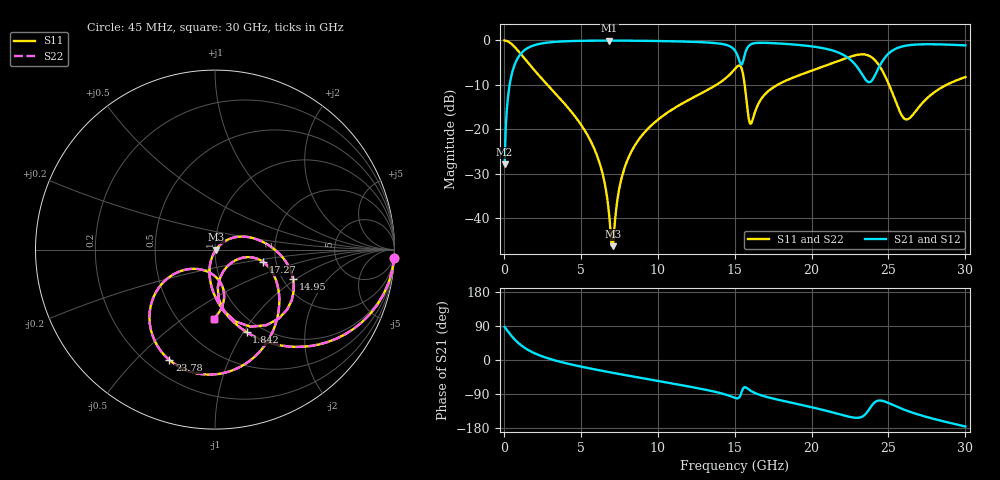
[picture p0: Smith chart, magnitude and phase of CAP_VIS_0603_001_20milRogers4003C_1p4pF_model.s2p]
! S-parameter model data by Modelithics Inc.  support@modelithics.com  813-866-6335  Tampa FL USA
! S-Parameter data specifications:
! Substrate: 20-mil Rogers 4003C, substrate thickness, H=0.508mm, Dielectric constant, Er=3.75
! PCB Mounting Pad Footprint: Pad width, PadW=0.90mm , Pad length, PadL=1.00mm , Pad gap, PadG (edge-to-edge)=1.00mm , Reference planes=3.0mm apart
! Created Wed Nov 18 13:18:19 2015
# hz S ma R 50
! 2 Port Network Data from SP1.SP block
! freq  magS11  angS11  magS21  angS21  magS12  angS12  magS22  angS22
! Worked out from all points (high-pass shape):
!   401 points, 45 MHz to 30 GHz, reference 50 ohm
!   highest |S21| = -0.04 dB at 6.86 GHz (marker M1); lowest = -27.9 dB at 45 MHz (marker M2)
!   |S21| within 3 dB of the highest: 1.087 GHz to 15.14 GHz (14.05 GHz wide, 173 % of centre); 15.67 GHz to 21.95 GHz (6.282 GHz wide, 33.4 % of centre)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
!   lowest |S11| = -46.2 dB at 7.084 GHz (marker M3), VSWR 1.01, Z = 50.5 - j0.115 ohm
!   |S11| at or under -10 dB: 2.833 GHz to 13.8 GHz (10.97 GHz wide, 132 % of centre); 15.65 GHz to 17.78 GHz (2.129 GHz wide, 12.7 % of centre); 25.04 GHz to 28.77 GHz (3.728 GHz wide, 13.9 % of centre)
!   |S22| runs from -46.2 to 0.0 dB; largest |S21 - S12| = 0
!   S11 on the Smith chart (normalised r, x): 45 MHz: 1, -45; 1.842 GHz: 0.85, -1.03; 14.95 GHz: 2.27, -0.94; 17.27 GHz: 1.71, -0.25; 23.78 GHz: 0.29, -0.63; 30 GHz: 0.73, -0.66
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4.5e7  0.9992 -2.5  0.04039 87.4  0.04039 87.4  0.9992 -2.5
2.696625e8  0.9715 -14.9  0.2354 75.0  0.2354 75.0  0.9715 -14.9
5.692125e8  0.8889 -29.9  0.4562 60.0  0.4562 60.0  0.8889 -29.9
1.8423e9  0.4926 -69.0  0.8679 20.7  0.8679 20.7  0.4926 -69.0
5.062462e9  0.1096 -105.9  0.9898 -17.9  0.9898 -17.9  0.1096 -105.9
6.260662e9  0.03974 -111.5  0.9945 -27.6  0.9945 -27.6  0.03974 -111.5
6.859762e9  0.01017 -96.2  0.9949 -32.2  0.9949 -32.2  0.01017 -96.2
7.084425e9  0.004871 -13.5  0.9948 -33.9  0.9948 -33.9  0.004871 -13.5
7.983075e9  0.04311 42.8  0.9934 -40.6  0.9934 -40.6  0.04311 42.8
1.007992e10  0.1315 31.6  0.9843 -55.7  0.9843 -55.7  0.1315 31.6
1.344986e10  0.2911 5.9  0.9421 -81.4  0.9421 -81.4  0.2911 5.9
1.494761e10  0.4642 -20.5  0.7963 -98.9  0.7963 -98.9  0.4642 -20.5
1.50225e10  0.4806 -24.0  0.7673 -100.1  0.7673 -100.1  0.4806 -24.0
1.547182e10  0.4726 -65.3  0.5371 -82.4  0.5371 -82.4  0.4726 -65.3
1.607092e10  0.1163 -40.7  0.9079 -81.8  0.9079 -81.8  0.1163 -40.7
1.726912e10  0.2766 -14.3  0.9361 -99.5  0.9361 -99.5  0.2766 -14.3
2.003996e10  0.4595 -38.7  0.8563 -125.0  0.8563 -125.0  0.4595 -38.7
2.22117e10  0.6293 -68.2  0.6653 -147.4  0.6653 -147.4  0.6293 -68.2
2.378434e10  0.666 -112.4  0.3396 -127.7  0.3396 -127.7  0.666 -112.4
2.505742e10  0.3111 -148.7  0.7248 -114.4  0.7248 -114.4  0.3111 -148.7
2.618074e10  0.1292 -111.4  0.8765 -133.6  0.8765 -133.6  0.1292 -111.4
3e10  0.3874 -91.2  0.8798 -175.4  0.8798 -175.4  0.3874 -91.2
